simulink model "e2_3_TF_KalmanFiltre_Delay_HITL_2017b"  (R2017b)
settings: Solver=ode4  StartTime=0.0  StopTime=100  FixedStep=sampleTime  RelTol=1e-3  EnableMultiTasking=on
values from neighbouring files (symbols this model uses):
  k_d_x = 0.7    [startSimulation.m]
  k_d_y = 0.7    [startSimulation.m]
  k_d_yaw = 0.05    [startSimulation.m]
  k_d_z = 0.05    [startSimulation.m]
  k_i_x = 0.01    [startSimulation.m]
  k_i_y = 0.01    [startSimulation.m]
  k_i_yaw = 0.01    [startSimulation.m]
  k_i_z = 0.01    [startSimulation.m]
  k_p_x = 1    [startSimulation.m]
  k_p_y = 1    [startSimulation.m]
  k_p_yaw = 2    [startSimulation.m]
  k_p_z = 3    [startSimulation.m]
  saturation_psi = 2    [startSimulation.m]
  saturation_x = 2    [startSimulation.m]
  saturation_y = 2    [startSimulation.m]
  saturation_z = 2    [startSimulation.m]
undefined symbols (not defined in the file or in its folder): DiscIntNeverNeededParam, KiRollAttitude, sigbuilder_block
libraries: simulink x10, aerolibanimutils x2, etargetslib x2
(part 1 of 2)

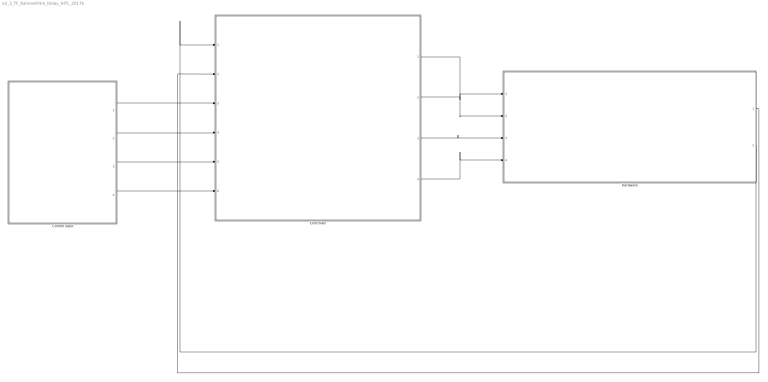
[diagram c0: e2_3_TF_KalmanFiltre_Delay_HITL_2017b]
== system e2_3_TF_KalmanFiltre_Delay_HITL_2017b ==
  Control Input : Subsystem
  "Controller " : Subsystem
  Hardware : Subsystem
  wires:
  "Controller "/1(Controller Output X) -> Hardware/1(X)
  "Controller "/2(Controller Output Y) -> Hardware/2(Y)
  "Controller "/3(Controller Output H) -> Hardware/3(H)
  "Controller "/4(Controller Output Psi) -> Hardware/4(Psi)
  Control Input/1(ux) -> "Controller "/3(Control input X)
  Control Input/2(uy) -> "Controller "/4(Control input Y)
  Control Input/3(uz) -> "Controller "/5(Control input H)
  Control Input/4(upsi) -> "Controller "/6(Control input Psi)
  Hardware/1(Vel) -> "Controller "/2(Feedback Velocity)
  Hardware/2(Pos) -> "Controller "/1(Feedback Position)

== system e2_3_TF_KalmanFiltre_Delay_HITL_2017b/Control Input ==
  Bloc Test Position Fixe : Subsystem
  Bus Creator : BusCreator  Inputs=4
  Demux : Demux
  Simulation Pace : aerolibanimutils/Simulation Pace  Commented=on  SimulationPace=100  SleepMode=MATLAB Thread  OutputPaceError=off  SampleTime=-1
  ux : Outport  VectorParamsAs1DForOutWhenUnconnected=off
  uy : Outport  Port=2  VectorParamsAs1DForOutWhenUnconnected=off
  uz : Outport  Port=3  VectorParamsAs1DForOutWhenUnconnected=off
  upsi : Outport  Port=4  VectorParamsAs1DForOutWhenUnconnected=off
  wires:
  Demux/2 -> uy/1
  Demux/1 -> ux/1
  Bloc Test Position Fixe/2(uy) -> Bus Creator/2
  Demux/3 -> uz/1
  Demux/4 -> upsi/1
  Bloc Test Position Fixe/4(upsi) -> Bus Creator/4
  Bloc Test Position Fixe/3(uz) -> Bus Creator/3
  Bloc Test Position Fixe/1(ux) -> Bus Creator/1
  Bus Creator/1 -> Demux/1

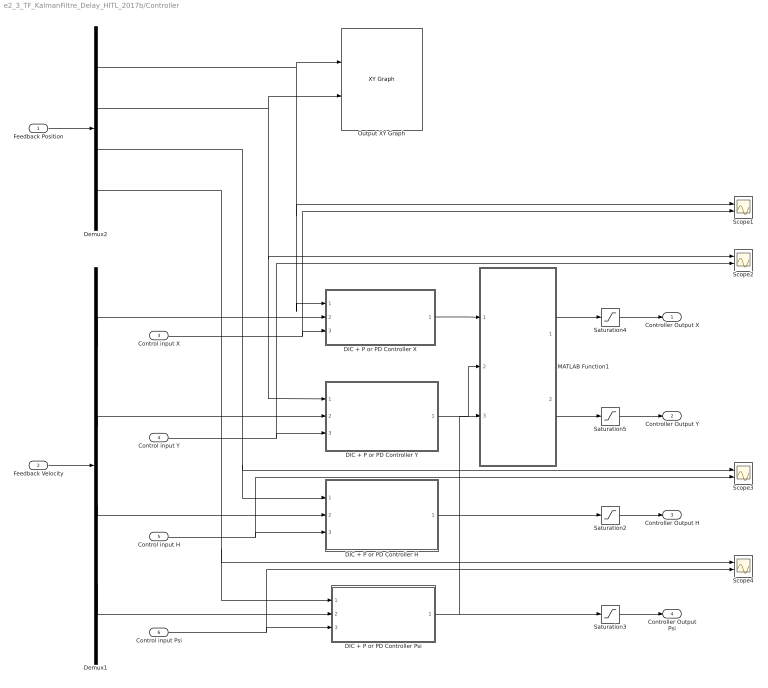
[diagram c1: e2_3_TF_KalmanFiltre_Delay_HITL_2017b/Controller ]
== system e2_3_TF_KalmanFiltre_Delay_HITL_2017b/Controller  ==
  Feedback Position : Inport
  Feedback Velocity : Inport  Port=2
  Control input X : Inport  Port=3
  Control input Y : Inport  Port=4
  Control input H : Inport  Port=5
  Control input Psi : Inport  Port=6
  DIC + P or PD Controller H : Subsystem
  DIC + P or PD Controller Psi : Subsystem
  DIC + P or PD Controller X : Subsystem
  DIC + P or PD Controller Y : Subsystem
  Demux1 : Demux
  Demux2 : Demux
  MATLAB Function1 : MATLAB Function  TreatAsAtomicUnit=on
  Output XY Graph : simulink/Sinks/XY Graph  Commented=on  xmin=-5  xmax=5  ymin=-5  ymax=5  st=-1
  Saturation2 : Saturate  UpperLimit=saturation_z  LowerLimit=-saturation_z
  Saturation3 : Saturate  UpperLimit=saturation_psi  LowerLimit=-saturation_psi
  Saturation4 : Saturate  UpperLimit=saturation_x  LowerLimit=-saturation_x
  Saturation5 : Saturate  UpperLimit=saturation_y  LowerLimit=-saturation_y
  Scope{1..4} (4 alike) : Scope  NumInputPorts=2
  Controller Output X : Outport  VectorParamsAs1DForOutWhenUnconnected=off
  Controller Output Y : Outport  Port=2  VectorParamsAs1DForOutWhenUnconnected=off
  Controller Output H : Outport  Port=3  VectorParamsAs1DForOutWhenUnconnected=off
  Controller Output Psi : Outport  Port=4  VectorParamsAs1DForOutWhenUnconnected=off
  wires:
  Feedback Position/1 -> Demux2/1
  Feedback Velocity/1 -> Demux1/1
  Demux1/2 -> DIC + P or PD Controller Y/2(Feedback Velocity Y)
  Demux2/3 -> Scope3/1, DIC + P or PD Controller H/1(Feedback Position H)
  Demux1/1 -> DIC + P or PD Controller X/2(Feedback Velocity X)
  Demux1/3 -> DIC + P or PD Controller H/2(Feedback Velocity H)
  Control input X/1 -> Scope1/2, DIC + P or PD Controller X/3(Control Input X)
  Control input H/1 -> Scope3/2, DIC + P or PD Controller H/3(Control Input H)
  Saturation4/1 -> Controller Output X/1
  Saturation5/1 -> Controller Output Y/1
  Saturation2/1 -> Controller Output H/1
  Saturation3/1 -> Controller Output Psi/1
  Control input Y/1 -> Scope2/2, DIC + P or PD Controller Y/3(Control Input Y)
  DIC + P or PD Controller H/1(Controller Output H) -> Saturation2/1
  DIC + P or PD Controller Psi/1(Controller Output Psi) -> MATLAB Function1/3(psi), Saturation3/1
  Demux2/1 -> Scope1/1, DIC + P or PD Controller X/1(Feedback Position X), Output XY Graph/1
  Demux2/2 -> Scope2/1, DIC + P or PD Controller Y/1(Feedback Position Y), Output XY Graph/2
  Demux2/4 -> Scope4/1, DIC + P or PD Controller Psi/1(Feedback Position Psi)
  Demux1/4 -> DIC + P or PD Controller Psi/2(Feedback Velocity Psi)
  Control input Psi/1 -> Scope4/2, DIC + P or PD Controller Psi/3(Control input Psi)
  MATLAB Function1/2(y) -> Saturation5/1
  MATLAB Function1/1(x) -> Saturation4/1
  DIC + P or PD Controller X/1(Controller Output X) -> MATLAB Function1/1(eax)
  DIC + P or PD Controller Y/1(Controller Output Y) -> MATLAB Function1/2(eay)

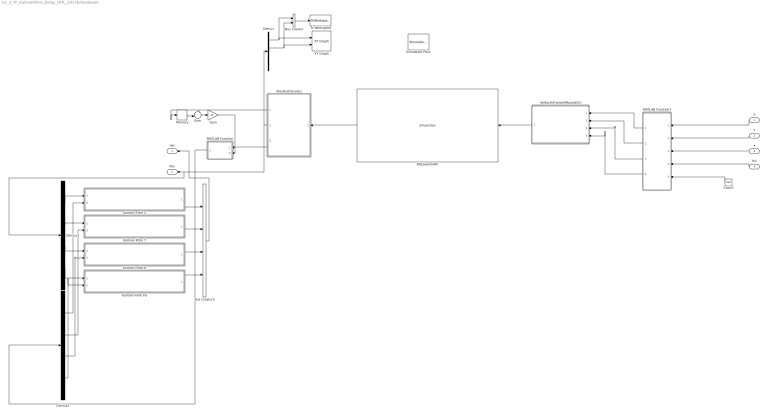
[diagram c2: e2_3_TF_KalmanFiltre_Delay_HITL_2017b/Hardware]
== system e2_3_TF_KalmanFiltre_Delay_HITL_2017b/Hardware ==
  X : Inport
  Y : Inport  Port=2
  H : Inport  Port=3
  Psi : Inport  Port=4
  Bus Creator : BusCreator  Inputs=2
  Bus Creator5 : BusCreator  Inputs=4
  Clock1 : Clock
  Demux : Demux
  Demux1 : Demux
  Demux2 : Demux
  Gain : Gain  Gain=25
  Kalman Filtre H : Subsystem
  Kalman Filtre Psi : Subsystem
  Kalman Filtre X : Subsystem
  Kalman Filtre Y : Subsystem
  MATLAB Function : MATLAB Function  TreatAsAtomicUnit=on
  MATLAB Function7 : MATLAB Function  TreatAsAtomicUnit=on
  MavOutDecode1 : MATLAB Function  TreatAsAtomicUnit=on
  Memory : Memory
  RflySwarmAPI : S-Function  FunctionName=RflyUdpFast  Parameters=port,num,modeValue,T,ip  SFunctionDeploymentMode=off  EnableBusSupport=off  mask(UDP Receive){ip=255.255.255.255, port=20100, num=1, mode=FullData Mode, T=1/25, modeValue=0}
      mask prompts: ip "UDP IP Address"; port "UDP Port"; num "vehicle Number"; mode "UDP Mode"; T "Sample Time"
      mask help: This block receives bytes from an UDP/IP connection. The first parameter is the UDP port on the first CopterSim App The second parameter is the total vehicle number The third parameter is the data mode. check the help button for the definition
      mask init:
      | if strcmp(mode,'FullData Mode')
      |     modeValue = 0;
      | elseif strcmp(mode,'SimpleData Mode') 
      |     modeValue = 1;
      | elseif strcmp(mode,'UltraSimple Mode') 
      |     modeValue = 2;
      | else
      |     modeValue = 0;
      | end
  Simulation Pace : aerolibanimutils/Simulation Pace  SimulationPace=1  SleepMode=MATLAB Thread  OutputPaceError=off  SampleTime=-1
  Sum : Sum  Inputs=+-|
  To Workspace : ToWorkspace  VariableName=Pos1  SaveFormat=Timeseries  SampleTime=-1
  VelEarthFrameOffboardCtrl : Subsystem
  XY Graph : simulink/Sinks/XY Graph  Commented=on  xmin=-1  xmax=1  ymin=-1  ymax=1  st=-1
  Vel : Outport  VectorParamsAs1DForOutWhenUnconnected=off
  Pos : Outport  Port=2  VectorParamsAs1DForOutWhenUnconnected=off
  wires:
  Gain/1 -> MATLAB Function/2(psi)
  Demux/2 -> Bus Creator/2, XY Graph/2
  Demux/1 -> Bus Creator/1, XY Graph/1
  Sum/1 -> Gain/1
  X/1 -> MATLAB Function7/1(X)
  MATLAB Function7/2(y1) -> VelEarthFrameOffboardCtrl/2(VeY_ms)
  MATLAB Function7/3(h1) -> VelEarthFrameOffboardCtrl/3(VeZ_ms)
  MATLAB Function7/1(x1) -> VelEarthFrameOffboardCtrl/1(VeX_ms)
  Clock1/1 -> MATLAB Function7/5(t)
  Memory/1 -> Sum/2
  MavOutDecode1/1(Psi) -> Memory/1, Sum/1
  RflySwarmAPI/1 -> MavOutDecode1/1(u)
  VelEarthFrameOffboardCtrl/1(Out1) -> RflySwarmAPI/1
  Bus Creator/1 -> To Workspace/1
  MavOutDecode1/3(localVel) -> MATLAB Function/1(v)
  MATLAB Function7/4(p1) -> VelEarthFrameOffboardCtrl/4(yawRate_rads)
  Y/1 -> MATLAB Function7/2(Y)
  H/1 -> MATLAB Function7/3(H)
  Psi/1 -> MATLAB Function7/4(Psi)
  Demux1/1 -> Kalman Filtre X/1(The system output: Position)
  Kalman Filtre X/1(Out velocity feedback) -> Bus Creator5/1
  MavOutDecode1/2(localPos) -> Demux1/1, Pos/1, Demux/1
  Kalman Filtre Psi/1(Out velocity feedback) -> Bus Creator5/4
  Demux2/2 -> Kalman Filtre Y/2(In2)
  Demux1/4 -> Kalman Filtre Psi/1(The system output: Position)
  Demux1/2 -> Kalman Filtre Y/1(The system output: Position)
  Demux2/4 -> Kalman Filtre Psi/2(In2)
  Demux1/3 -> Kalman Filtre H/1(The system output: Position)
  Demux2/1 -> Kalman Filtre X/2(In2)
  Kalman Filtre H/1(Out velocity feedback) -> Bus Creator5/3
  MATLAB Function/1(y) -> Demux2/1
  Demux2/3 -> Kalman Filtre H/2(In2)
  Kalman Filtre Y/1(Out velocity feedback) -> Bus Creator5/2
  Bus Creator5/1 -> Vel/1

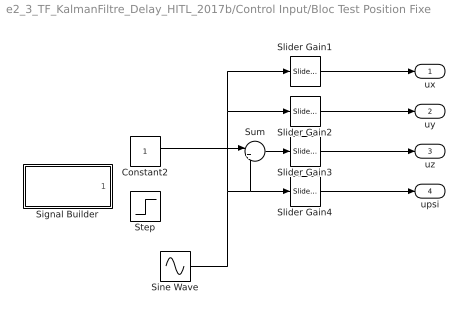
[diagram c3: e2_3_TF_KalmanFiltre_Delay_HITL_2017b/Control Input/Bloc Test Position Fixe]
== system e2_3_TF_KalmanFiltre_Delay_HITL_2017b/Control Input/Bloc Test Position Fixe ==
  Constant2 : Constant
  Signal Builder : Subsystem  Tag=STV Subsys  LoadFcn=sigbuilder_block('load');  StartFcn=sigbuilder_block('start');  StopFcn=sigbuilder_block('stop');  ClipboardFcn=sigbuilder_block('clipboard');  mask(Sigbuilder block){tuvar=[0:10]}
      mask help: Simulink:masks:SigbuilderBlock_MD
      mask init:
      | if ~strcmp(get_param(bdroot(gcbh),'SimulationStatus'),'stopped') tuvar = sigbuilder_block('maskInit'); end
  Sine Wave : Sin  Frequency=0.5  SampleTime=0
  Slider Gain1 : simulink/Math Operations/Slider Gain  gain=0  low=-10  high=10
  Slider Gain2 : simulink/Math Operations/Slider Gain  gain=0  low=-10  high=10
  Slider Gain3 : simulink/Math Operations/Slider Gain  gain=1  low=-2  high=2
  Slider Gain4 : simulink/Math Operations/Slider Gain  gain=0  low=-2  high=2
  Step : Step  Time=5  SampleTime=0
  Sum : Sum  Inputs=|++
  ux : Outport  VectorParamsAs1DForOutWhenUnconnected=off
  uy : Outport  Port=2  VectorParamsAs1DForOutWhenUnconnected=off
  uz : Outport  Port=3  VectorParamsAs1DForOutWhenUnconnected=off
  upsi : Outport  Port=4  VectorParamsAs1DForOutWhenUnconnected=off
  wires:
  Slider Gain1/1 -> ux/1
  Slider Gain2/1 -> uy/1
  Slider Gain3/1 -> uz/1
  Slider Gain4/1 -> upsi/1
  Constant2/1 -> Sum/1
  Sine Wave/1 -> Sum/2, Slider Gain4/1, Slider Gain2/1, Slider Gain1/1
  Sum/1 -> Slider Gain3/1

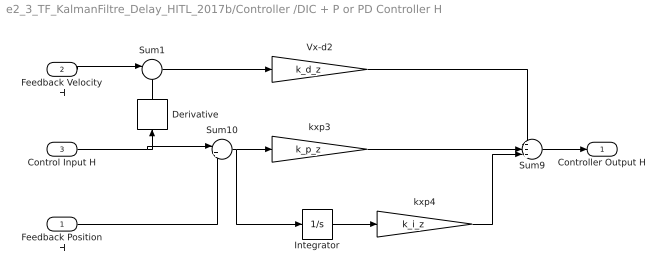
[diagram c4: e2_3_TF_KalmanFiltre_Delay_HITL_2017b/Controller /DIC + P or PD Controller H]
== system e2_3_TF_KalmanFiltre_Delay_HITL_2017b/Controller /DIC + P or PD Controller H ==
  Feedback Position H : Inport
  Feedback Velocity H : Inport  Port=2
  Control Input H : Inport  Port=3
  Derivative : Derivative
  Integrator : Integrator
  Sum1 : Sum  Inputs=|-+
  Sum10 : Sum  Inputs=|+-
  Sum9 : Sum  Inputs=+++|
  Vx-d2 : Gain  Gain=k_d_z
  kxp3 : Gain  Gain=k_p_z
  kxp4 : Gain  Gain=k_i_z
  Controller Output H : Outport  VectorParamsAs1DForOutWhenUnconnected=off
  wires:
  Sum9/1 -> Controller Output H/1
  Sum10/1 -> kxp3/1, Integrator/1
  kxp3/1 -> Sum9/2
  Vx-d2/1 -> Sum9/1
  Feedback Velocity H/1 -> Sum1/1
  Sum1/1 -> Vx-d2/1
  Integrator/1 -> kxp4/1
  kxp4/1 -> Sum9/3
  Control Input H/1 -> Sum10/1, Derivative/1
  Feedback Position H/1 -> Sum10/2
  Derivative/1 -> Sum1/2

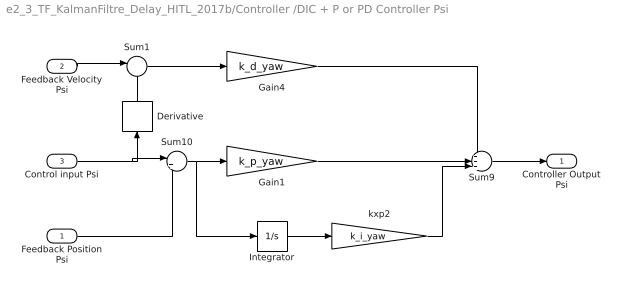
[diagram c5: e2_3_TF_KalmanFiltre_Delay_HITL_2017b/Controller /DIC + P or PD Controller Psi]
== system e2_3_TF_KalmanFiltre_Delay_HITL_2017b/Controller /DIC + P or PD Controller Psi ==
  Feedback Position Psi : Inport
  Feedback Velocity Psi : Inport  Port=2
  Control input Psi : Inport  Port=3
  Derivative : Derivative
  Gain1 : Gain  Gain=k_p_yaw
  Gain4 : Gain  Gain=k_d_yaw
  Integrator : Integrator
  Sum1 : Sum  Inputs=|-+
  Sum10 : Sum  Inputs=|+-
  Sum9 : Sum  Inputs=+++|
  kxp2 : Gain  Gain=k_i_yaw
  Controller Output Psi : Outport  VectorParamsAs1DForOutWhenUnconnected=off
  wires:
  Sum9/1 -> Controller Output Psi/1
  kxp2/1 -> Sum9/3
  Control input Psi/1 -> Sum10/1, Derivative/1
  Gain4/1 -> Sum9/1
  Sum10/1 -> Gain1/1, Integrator/1
  Integrator/1 -> kxp2/1
  Feedback Velocity Psi/1 -> Sum1/1
  Sum1/1 -> Gain4/1
  Gain1/1 -> Sum9/2
  Derivative/1 -> Sum1/2
  Feedback Position Psi/1 -> Sum10/2

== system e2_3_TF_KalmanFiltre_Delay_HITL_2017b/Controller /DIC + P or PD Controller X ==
  Feedback Position X : Inport
  Feedback Velocity X : Inport  Port=2
  Control Input X : Inport  Port=3
  PID1 : Subsystem
  Sum3 : Sum  Inputs=|+-
  Sum4 : Sum  Inputs=|+-
  roll_attitude2 : simulink/Continuous/PID Controller  Controller=P  Form=Parallel  TimeDomain=Discrete-time  SampleTime=-1  IntegratorMethod=Forward Euler  FilterMethod=Forward Euler  ControllerParametersSource=internal  P=1  I=KiRollAttitude  D=0.01  UseFilter=on  N=100  TunerSelectOption=Transfer Function Based (PID Tuner App)  InitialConditionSource=internal  InitialConditionForIntegrator=0  InitialConditionForFilter=0  DifferentiatorICPrevScaledInput=0  ExternalReset=none  TrackingMode=off  Kt=1  LimitOutput=on  UpperSaturationLimit=100  LowerSaturationLimit=-100  LinearizeAsGain=on  AntiWindupMode=back-calculation  Kb=1  POutMin=[]  POutMax=[]  IOutMin=[]  IOutMax=[]  DOutMin=[]  DOutMax=[]  NOutMin=[]  NOutMax=[]  SumOutMin=[]  SumOutMax=[]  SaturationOutMin=[]  SaturationOutMax=[]  PParamMin=[]  PParamMax=[]  IParamMin=[]  IParamMax=[]  DParamMin=[]  DParamMax=[]  NParamMin=[]  NParamMax=[]  KbParamMin=[]  KbParamMax=[]  KtParamMin=[]  KtParamMax=[]  KbOutMin=[]  KbOutMax=[]  KtOutMin=[]  KtOutMax=[]  IntegratorOutMin=[]  IntegratorOutMax=[]  FilterOutMin=[]  FilterOutMax=[]  SumI1OutMin=[]  SumI1OutMax=[]  SumI2OutMin=[]  SumI2OutMax=[]  SumI3OutMin=[]  SumI3OutMax=[]  SumDOutMin=[]  SumDOutMax=[]  DifferentiatorOutMin=[]  DifferentiatorOutMax=[]  FilterDiffOutCoefMin=[]  FilterDiffOutCoefMax=[]  ReciprocalOutMin=[]  ReciprocalOutMax=[]  SumDenOutMin=[]  SumDenOutMax=[]  SumNumOutMin=[]  SumNumOutMax=[]  DivideOutMin=[]  DivideOutMax=[]  IntegratorContinuousStateAttributes=''  IntegratorStateMustResolveToSignalObject=off  IntegratorRTWStateStorageClass=Auto  FilterContinuousStateAttributes=''  FilterStateMustResolveToSignalObject=off  FilterRTWStateStorageClass=Auto  InitialConditionSetting=State (most efficient)
  Controller Output X : Outport  VectorParamsAs1DForOutWhenUnconnected=off
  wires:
  roll_attitude2/1 -> Sum4/1
  Sum3/1 -> roll_attitude2/1
  Sum4/1 -> PID1/1(x)
  PID1/1(y) -> Controller Output X/1
  Feedback Velocity X/1 -> Sum4/2
  Control Input X/1 -> Sum3/1
  Feedback Position X/1 -> Sum3/2

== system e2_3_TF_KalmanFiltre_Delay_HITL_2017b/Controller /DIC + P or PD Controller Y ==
  Feedback Position Y : Inport
  Feedback Velocity Y : Inport  Port=2
  Control Input Y : Inport  Port=3
  PID2 : Subsystem
  Sum : Sum  Inputs=|+-
  Sum2 : Sum  Inputs=|+-
  roll_attitude : simulink/Continuous/PID Controller  Controller=P  Form=Parallel  TimeDomain=Discrete-time  SampleTime=-1  IntegratorMethod=Forward Euler  FilterMethod=Forward Euler  ControllerParametersSource=internal  P=1  I=KiRollAttitude  D=0.01  UseFilter=on  N=100  TunerSelectOption=Transfer Function Based (PID Tuner App)  InitialConditionSource=internal  InitialConditionForIntegrator=0  InitialConditionForFilter=0  DifferentiatorICPrevScaledInput=0  ExternalReset=none  TrackingMode=off  Kt=1  LimitOutput=on  UpperSaturationLimit=1  LowerSaturationLimit=-1  LinearizeAsGain=on  AntiWindupMode=back-calculation  Kb=1  POutMin=[]  POutMax=[]  IOutMin=[]  IOutMax=[]  DOutMin=[]  DOutMax=[]  NOutMin=[]  NOutMax=[]  SumOutMin=[]  SumOutMax=[]  SaturationOutMin=[]  SaturationOutMax=[]  PParamMin=[]  PParamMax=[]  IParamMin=[]  IParamMax=[]  DParamMin=[]  DParamMax=[]  NParamMin=[]  NParamMax=[]  KbParamMin=[]  KbParamMax=[]  KtParamMin=[]  KtParamMax=[]  KbOutMin=[]  KbOutMax=[]  KtOutMin=[]  KtOutMax=[]  IntegratorOutMin=[]  IntegratorOutMax=[]  FilterOutMin=[]  FilterOutMax=[]  SumI1OutMin=[]  SumI1OutMax=[]  SumI2OutMin=[]  SumI2OutMax=[]  SumI3OutMin=[]  SumI3OutMax=[]  SumDOutMin=[]  SumDOutMax=[]  DifferentiatorOutMin=[]  DifferentiatorOutMax=[]  FilterDiffOutCoefMin=[]  FilterDiffOutCoefMax=[]  ReciprocalOutMin=[]  ReciprocalOutMax=[]  SumDenOutMin=[]  SumDenOutMax=[]  SumNumOutMin=[]  SumNumOutMax=[]  DivideOutMin=[]  DivideOutMax=[]  IntegratorContinuousStateAttributes=''  IntegratorStateMustResolveToSignalObject=off  IntegratorRTWStateStorageClass=Auto  FilterContinuousStateAttributes=''  FilterStateMustResolveToSignalObject=off  FilterRTWStateStorageClass=Auto  InitialConditionSetting=State (most efficient)
  Controller Output Y : Outport  VectorParamsAs1DForOutWhenUnconnected=off
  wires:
  Sum/1 -> roll_attitude/1
  roll_attitude/1 -> Sum2/1
  Sum2/1 -> PID2/1(x)
  Feedback Position Y/1 -> Sum/2
  Feedback Velocity Y/1 -> Sum2/2
  Control Input Y/1 -> Sum/1
  PID2/1(y) -> Controller Output Y/1

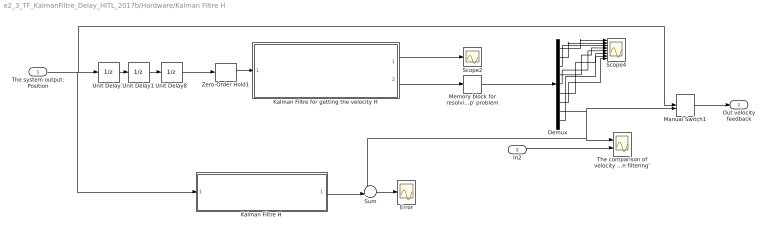
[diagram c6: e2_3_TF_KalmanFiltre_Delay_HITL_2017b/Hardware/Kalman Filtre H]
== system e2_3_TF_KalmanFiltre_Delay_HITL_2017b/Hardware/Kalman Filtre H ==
  The system output: Position : Inport
  In2 : Inport  Port=2
  Demux : Demux  Outputs=9
  Error : Scope
  Kalman Filtre H : Subsystem
  Kalman Filtre for getting the velocity H : MATLAB Function  TreatAsAtomicUnit=on
  Manual Switch1 : ManualSwitch  CurrentSetting=0
  Memory block for resolving the 'algebraic loop' problem : Memory
  Scope2 : Scope
  Scope4 : Scope  NumInputPorts=8
  Sum : Sum  Inputs=-+|
  The comparison of velocity signal between 'Derivative' and 'Kalman filtering' : Scope  NumInputPorts=2
  Unit Delay1 : UnitDelay  SampleTime=-1  HasFrameUpgradeWarning=on
  Unit Delay7 : UnitDelay  SampleTime=-1  HasFrameUpgradeWarning=on
  Unit Delay8 : UnitDelay  SampleTime=-1  HasFrameUpgradeWarning=on
  Zero-Order Hold1 : ZeroOrderHold  SampleTime=-1
  Out velocity feedback : Outport  VectorParamsAs1DForOutWhenUnconnected=off
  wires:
  Kalman Filtre for getting the velocity H/1(Covariance_matrice) -> Scope2/1
  Kalman Filtre for getting the velocity H/2(X_Kalmanfiltred) -> Memory block for resolving the 'algebraic loop' problem/1
  Memory block for resolving the 'algebraic loop' problem/1 -> Demux/1
  Zero-Order Hold1/1 -> Kalman Filtre for getting the velocity H/1(Mesurement_Velocity)
  Manual Switch1/1 -> Out velocity feedback/1
  Demux/1 -> Scope4/1
  The system output: Position/1 -> Kalman Filtre H/1(The system output: Position), Manual Switch1/1, Unit Delay7/1
  Demux/2 -> Scope4/2
  Demux/3 -> Scope4/3
  Demux/4 -> Scope4/4
  Demux/5 -> Scope4/5
  Unit Delay8/1 -> Zero-Order Hold1/1
  Demux/6 -> Scope4/6
  Demux/7 -> Scope4/8
  Demux/8 -> Sum/1, The comparison of velocity signal between 'Derivative' and 'Kalman filtering'/1, Manual Switch1/2
  Demux/9 -> Scope4/7
  In2/1 -> The comparison of velocity signal between 'Derivative' and 'Kalman filtering'/2
  Unit Delay7/1 -> Unit Delay1/1
  Unit Delay1/1 -> Unit Delay8/1
  Sum/1 -> Error/1
  Kalman Filtre H/1(Out velocity feedback) -> Sum/2

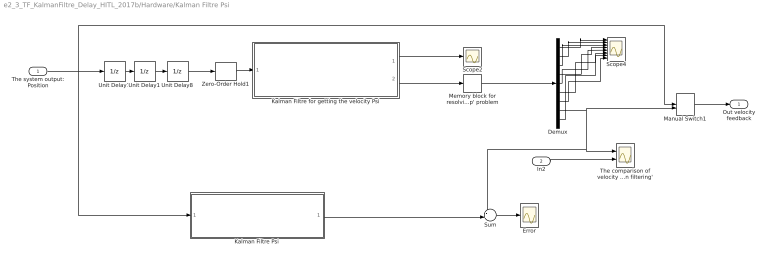
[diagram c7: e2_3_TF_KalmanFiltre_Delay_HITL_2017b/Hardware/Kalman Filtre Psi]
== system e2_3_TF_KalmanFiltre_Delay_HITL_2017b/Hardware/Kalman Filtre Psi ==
  The system output: Position : Inport
  In2 : Inport  Port=2
  Demux : Demux  Outputs=9
  Error : Scope
  Kalman Filtre Psi : Subsystem
  Kalman Filtre for getting the velocity Psi : MATLAB Function  TreatAsAtomicUnit=on
  Manual Switch1 : ManualSwitch  CurrentSetting=0
  Memory block for resolving the 'algebraic loop' problem : Memory
  Scope2 : Scope
  Scope4 : Scope  NumInputPorts=8
  Sum : Sum  Inputs=-+|
  The comparison of velocity signal between 'Derivative' and 'Kalman filtering' : Scope  NumInputPorts=2
  Unit Delay1 : UnitDelay  SampleTime=-1  HasFrameUpgradeWarning=on
  Unit Delay7 : UnitDelay  SampleTime=-1  HasFrameUpgradeWarning=on
  Unit Delay8 : UnitDelay  SampleTime=-1  HasFrameUpgradeWarning=on
  Zero-Order Hold1 : ZeroOrderHold  SampleTime=-1
  Out velocity feedback : Outport  VectorParamsAs1DForOutWhenUnconnected=off
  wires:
  Kalman Filtre for getting the velocity Psi/1(Covariance_matrice) -> Scope2/1
  Kalman Filtre for getting the velocity Psi/2(X_Kalmanfiltred) -> Memory block for resolving the 'algebraic loop' problem/1
  Memory block for resolving the 'algebraic loop' problem/1 -> Demux/1
  Zero-Order Hold1/1 -> Kalman Filtre for getting the velocity Psi/1(Mesurement_Velocity)
  Manual Switch1/1 -> Out velocity feedback/1
  Demux/1 -> Scope4/1
  The system output: Position/1 -> Kalman Filtre Psi/1(The system output: Position), Manual Switch1/1, Unit Delay7/1
  Demux/2 -> Scope4/2
  Demux/3 -> Scope4/3
  Demux/4 -> Scope4/4
  Demux/5 -> Scope4/5
  Unit Delay8/1 -> Zero-Order Hold1/1
  Demux/6 -> Scope4/6
  Demux/7 -> Scope4/8
  Demux/8 -> Sum/1, The comparison of velocity signal between 'Derivative' and 'Kalman filtering'/1, Manual Switch1/2
  Demux/9 -> Scope4/7
  In2/1 -> The comparison of velocity signal between 'Derivative' and 'Kalman filtering'/2
  Unit Delay7/1 -> Unit Delay1/1
  Unit Delay1/1 -> Unit Delay8/1
  Sum/1 -> Error/1
  Kalman Filtre Psi/1(Out velocity feedback) -> Sum/2

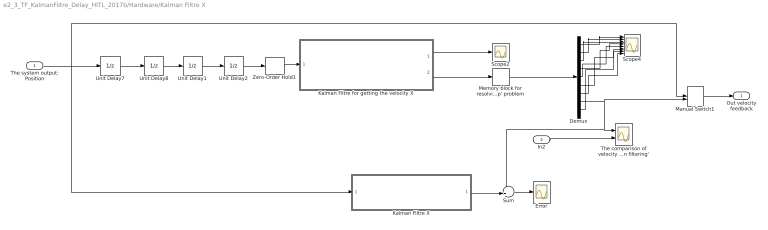
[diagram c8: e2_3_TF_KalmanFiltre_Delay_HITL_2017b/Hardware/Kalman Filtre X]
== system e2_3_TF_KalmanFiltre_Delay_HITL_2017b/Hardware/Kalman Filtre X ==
  The system output: Position : Inport
  In2 : Inport  Port=2
  Demux : Demux  Outputs=9
  Error : Scope
  Kalman Filtre X : Subsystem
  Kalman Filtre for getting the velocity X : MATLAB Function  TreatAsAtomicUnit=on
  Manual Switch1 : ManualSwitch  CurrentSetting=0
  Memory block for resolving the 'algebraic loop' problem : Memory  InheritSampleTime=on
  Scope2 : Scope
  Scope4 : Scope  NumInputPorts=8
  Sum : Sum  Inputs=-+|
  The comparison of velocity signal between 'Derivative' and 'Kalman filtering' : Scope  NumInputPorts=2
  Unit Delay{1..2,7..8} (4 alike) : UnitDelay  SampleTime=-1  HasFrameUpgradeWarning=on
  Zero-Order Hold1 : ZeroOrderHold  SampleTime=-1
  Out velocity feedback : Outport  VectorParamsAs1DForOutWhenUnconnected=off
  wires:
  Kalman Filtre for getting the velocity X/1(Covariance_matrice) -> Scope2/1
  Kalman Filtre for getting the velocity X/2(X_Kalmanfiltred) -> Memory block for resolving the 'algebraic loop' problem/1
  Memory block for resolving the 'algebraic loop' problem/1 -> Demux/1
  Zero-Order Hold1/1 -> Kalman Filtre for getting the velocity X/1(Mesurement_Velocity)
  Manual Switch1/1 -> Out velocity feedback/1
  Demux/1 -> Scope4/1
  The system output: Position/1 -> Kalman Filtre X/1(The system output: Position), Manual Switch1/1, Unit Delay7/1
  Demux/2 -> Scope4/2
  Demux/3 -> Scope4/3
  Demux/4 -> Scope4/4
  Demux/5 -> Scope4/5
  Unit Delay7/1 -> Unit Delay8/1
  Unit Delay8/1 -> Unit Delay1/1
  Demux/6 -> Scope4/6
  Demux/7 -> Scope4/8
  Demux/8 -> Sum/1, The comparison of velocity signal between 'Derivative' and 'Kalman filtering'/1, Manual Switch1/2
  Demux/9 -> Scope4/7
  In2/1 -> The comparison of velocity signal between 'Derivative' and 'Kalman filtering'/2
  Unit Delay1/1 -> Unit Delay2/1
  Unit Delay2/1 -> Zero-Order Hold1/1
  Kalman Filtre X/1(Out velocity feedback) -> Sum/2
  Sum/1 -> Error/1

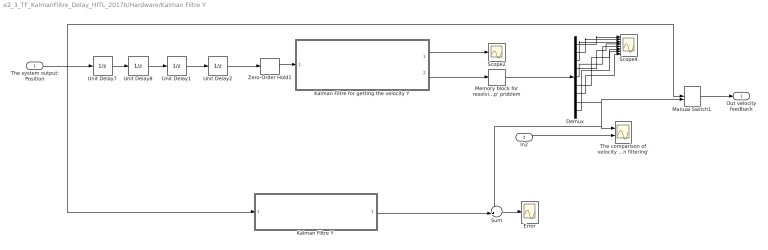
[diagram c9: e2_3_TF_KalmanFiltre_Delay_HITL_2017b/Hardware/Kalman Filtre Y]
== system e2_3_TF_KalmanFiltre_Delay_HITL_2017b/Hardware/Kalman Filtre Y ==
  The system output: Position : Inport
  In2 : Inport  Port=2
  Demux : Demux  Outputs=9
  Error : Scope
  Kalman Filtre Y : Subsystem
  Kalman Filtre for getting the velocity Y : MATLAB Function  TreatAsAtomicUnit=on
  Manual Switch1 : ManualSwitch  CurrentSetting=0
  Memory block for resolving the 'algebraic loop' problem : Memory
  Scope2 : Scope
  Scope4 : Scope  NumInputPorts=8
  Sum : Sum  Inputs=-+|
  The comparison of velocity signal between 'Derivative' and 'Kalman filtering' : Scope  NumInputPorts=2
  Unit Delay{1..2,7..8} (4 alike) : UnitDelay  SampleTime=-1  HasFrameUpgradeWarning=on
  Zero-Order Hold1 : ZeroOrderHold  SampleTime=-1
  Out velocity feedback : Outport  VectorParamsAs1DForOutWhenUnconnected=off
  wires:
  Kalman Filtre for getting the velocity Y/1(Covariance_matrice) -> Scope2/1
  Kalman Filtre for getting the velocity Y/2(X_Kalmanfiltred) -> Memory block for resolving the 'algebraic loop' problem/1
  Memory block for resolving the 'algebraic loop' problem/1 -> Demux/1
  Zero-Order Hold1/1 -> Kalman Filtre for getting the velocity Y/1(Mesurement_Velocity)
  Manual Switch1/1 -> Out velocity feedback/1
  Demux/1 -> Scope4/1
  The system output: Position/1 -> Kalman Filtre Y/1(The system output: Position), Unit Delay7/1, Manual Switch1/1
  Demux/2 -> Scope4/2
  Demux/3 -> Scope4/3
  Demux/4 -> Scope4/4
  Demux/5 -> Scope4/5
  Unit Delay2/1 -> Zero-Order Hold1/1
  Demux/6 -> Scope4/6
  Demux/7 -> Scope4/8
  Demux/8 -> Sum/1, The comparison of velocity signal between 'Derivative' and 'Kalman filtering'/1, Manual Switch1/2
  Demux/9 -> Scope4/7
  In2/1 -> The comparison of velocity signal between 'Derivative' and 'Kalman filtering'/2
  Unit Delay1/1 -> Unit Delay2/1
  Unit Delay8/1 -> Unit Delay1/1
  Unit Delay7/1 -> Unit Delay8/1
  Sum/1 -> Error/1
  Kalman Filtre Y/1(Out velocity feedback) -> Sum/2

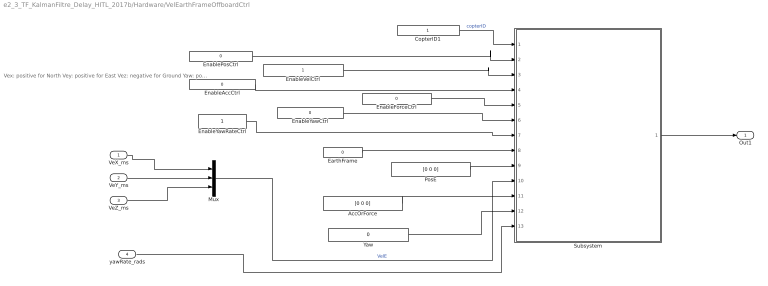
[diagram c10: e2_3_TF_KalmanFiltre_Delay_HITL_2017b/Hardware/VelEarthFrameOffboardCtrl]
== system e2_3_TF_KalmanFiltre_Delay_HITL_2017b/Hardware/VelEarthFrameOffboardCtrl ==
  note: Vex: positive for North Vey: positive for East Vez: negative for Ground Yaw: positive for right rotation
  VeX_ms : Inport
  VeY_ms : Inport  Port=2
  VeZ_ms : Inport  Port=3
  yawRate_rads : Inport  Port=4  PortDimensions=1
  AccOrForce : Constant  Value=[0 0 0]
  CopterID1 : Constant
  EarthFrame : Constant  Value=0
  EnableAccCtrl : Constant  Value=0
  EnableForceCtrl : Constant  Value=0
  EnablePosCtrl : Constant  Value=0
  EnableVelCtrl : Constant
  EnableYawCtrl : Constant  Value=0
  EnableYawRateCtrl : Constant
  Mux : Mux  Inputs=3
  PosE : Constant  Value=[0 0 0]
  Subsystem : Subsystem
  Yaw : Constant  Value=0
  Out1 : Outport
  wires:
  Yaw/1 -> Subsystem/12(yaw)
  EnableYawRateCtrl/1 -> Subsystem/7(EnYawrate)
  EnableYawCtrl/1 -> Subsystem/6(enYaw)
  EnableAccCtrl/1 -> Subsystem/4(enAcc)
  Mux/1 -> Subsystem/10(vel)  "VelE"
  EarthFrame/1 -> Subsystem/8(FrameIndex)
  yawRate_rads/1 -> Subsystem/13(yawrate)
  AccOrForce/1 -> Subsystem/11(acc)
  EnableVelCtrl/1 -> Subsystem/3(enVel)
  EnableForceCtrl/1 -> Subsystem/5(enForce)
  CopterID1/1 -> Subsystem/1(CopterID)  "copterID"
  EnablePosCtrl/1 -> Subsystem/2(enPos)
  PosE/1 -> Subsystem/9(pos)
  VeY_ms/1 -> Mux/2
  VeX_ms/1 -> Mux/1
  VeZ_ms/1 -> Mux/3
  Subsystem/1(Out1) -> Out1/1

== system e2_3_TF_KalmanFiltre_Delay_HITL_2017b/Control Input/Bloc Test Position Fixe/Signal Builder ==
  Demux : Demux  Tag=STV Demux  Outputs=1
  FromWs : FromWorkspace  Tag=STV FromWs  VariableName=tuvar
  Signal 2 : Outport  Tag=STV Outport  VectorParamsAs1DForOutWhenUnconnected=off
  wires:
  FromWs/1 -> Demux/1
  Demux/1 -> Signal 2/1

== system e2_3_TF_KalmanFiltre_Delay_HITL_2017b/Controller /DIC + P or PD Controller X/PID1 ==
  x : Inport
  Discrete Derivative : simulink/Discrete/Discrete Derivative  gainval=1.0  ICPrevScaledInput=0.0  OutMin=-5  OutMax=5  OutDataType=fixdt(1, 16)  OutScaling=2^-10  DoSatur=off
  Discrete-Time Integrator : DiscreteIntegrator  InitialConditionSetting=State (most efficient)  SampleTime=-1  LimitOutput=on  UpperSaturationLimit=5  LowerSaturationLimit=-5  ICPrevOutput=DiscIntNeverNeededParam  ICPrevScaledInput=DiscIntNeverNeededParam
  Sum : Sum  Inputs=+++  OutMin=-10  OutMax=10
  Vx-d3 : Gain  Gain=k_d_x
  kxp2 : Gain  Gain=k_i_x
  kxp3 : Gain  Gain=k_p_x
  y : Outport  InitialOutput=0  VectorParamsAs1DForOutWhenUnconnected=off
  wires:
  x/1 -> Vx-d3/1, kxp2/1, kxp3/1
  kxp2/1 -> Discrete-Time Integrator/1
  Vx-d3/1 -> Discrete Derivative/1
  kxp3/1 -> Sum/1
  Sum/1 -> y/1
  Discrete Derivative/1 -> Sum/3
  Discrete-Time Integrator/1 -> Sum/2

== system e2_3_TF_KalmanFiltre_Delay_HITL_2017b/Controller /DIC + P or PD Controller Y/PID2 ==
  x : Inport
  Discrete Derivative : simulink/Discrete/Discrete Derivative  gainval=1.0  ICPrevScaledInput=0.0  OutMin=[]  OutMax=[]  OutDataType=fixdt(1, 16)  OutScaling=2^-10  DoSatur=off
  Discrete-Time Integrator : DiscreteIntegrator  InitialConditionSetting=State (most efficient)  SampleTime=-1  LimitOutput=on  UpperSaturationLimit=10  LowerSaturationLimit=-10  ICPrevOutput=DiscIntNeverNeededParam  ICPrevScaledInput=DiscIntNeverNeededParam
  Sum : Sum  Inputs=+++  OutMin=-10  OutMax=10
  Vx-d2 : Gain  Gain=k_d_y
  kxp2 : Gain  Gain=k_p_y
  kxp3 : Gain  Gain=k_i_y
  y : Outport  InitialOutput=0  VectorParamsAs1DForOutWhenUnconnected=off
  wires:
  x/1 -> kxp2/1, kxp3/1, Vx-d2/1
  kxp3/1 -> Discrete-Time Integrator/1
  Vx-d2/1 -> Discrete Derivative/1
  kxp2/1 -> Sum/1
  Sum/1 -> y/1
  Discrete Derivative/1 -> Sum/3
  Discrete-Time Integrator/1 -> Sum/2

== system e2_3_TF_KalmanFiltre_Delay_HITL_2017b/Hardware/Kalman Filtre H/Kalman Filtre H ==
  The system output: Position : Inport
  Demux : Demux  Outputs=3
  Kalman Filtre for getting the velocity H : MATLAB Function  TreatAsAtomicUnit=on
  Memory block for resolving the 'algebraic loop' problem : Memory
  Scope2 : Scope
  Scope4 : Scope  NumInputPorts=2
  Out velocity feedback : Outport  VectorParamsAs1DForOutWhenUnconnected=off
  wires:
  Demux/2 -> Out velocity feedback/1
  Memory block for resolving the 'algebraic loop' problem/1 -> Demux/1
  Kalman Filtre for getting the velocity H/1(Covariance_matrice) -> Scope2/1
  The system output: Position/1 -> Kalman Filtre for getting the velocity H/1(Mesurement_Velocity)
  Demux/1 -> Scope4/1
  Kalman Filtre for getting the velocity H/2(X_Kalmanfiltred) -> Memory block for resolving the 'algebraic loop' problem/1
  Demux/3 -> Scope4/2

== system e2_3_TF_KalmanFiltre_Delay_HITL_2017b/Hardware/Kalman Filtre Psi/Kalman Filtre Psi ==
  The system output: Position : Inport
  Demux : Demux  Outputs=3
  Kalman Filtre for getting the velocity Psi : MATLAB Function  TreatAsAtomicUnit=on
  Memory block for resolving the 'algebraic loop' problem : Memory
  Scope1 : Scope  NumInputPorts=2
  Scope2 : Scope
  Out velocity feedback : Outport  VectorParamsAs1DForOutWhenUnconnected=off
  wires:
  Demux/2 -> Out velocity feedback/1
  Kalman Filtre for getting the velocity Psi/1(Covariance_matrice) -> Scope2/1
  The system output: Position/1 -> Kalman Filtre for getting the velocity Psi/1(Mesurement_Velocity)
  Demux/1 -> Scope1/1
  Demux/3 -> Scope1/2
  Kalman Filtre for getting the velocity Psi/2(X_Kalmanfiltred) -> Memory block for resolving the 'algebraic loop' problem/1
  Memory block for resolving the 'algebraic loop' problem/1 -> Demux/1

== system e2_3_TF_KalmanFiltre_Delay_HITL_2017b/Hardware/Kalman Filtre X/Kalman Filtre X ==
  The system output: Position : Inport
  Demux : Demux  Outputs=3
  Kalman Filtre for getting the velocity X : MATLAB Function  TreatAsAtomicUnit=on
  Memory block for resolving the 'algebraic loop' problem : Memory
  Scope2 : Scope
  Scope4 : Scope  NumInputPorts=2
  Out velocity feedback : Outport  VectorParamsAs1DForOutWhenUnconnected=off
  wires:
  Kalman Filtre for getting the velocity X/1(Covariance_matrice) -> Scope2/1
  Kalman Filtre for getting the velocity X/2(X_Kalmanfiltred) -> Memory block for resolving the 'algebraic loop' problem/1
  Memory block for resolving the 'algebraic loop' problem/1 -> Demux/1
  The system output: Position/1 -> Kalman Filtre for getting the velocity X/1(Mesurement_Velocity)
  Demux/2 -> Out velocity feedback/1
  Demux/1 -> Scope4/2
  Demux/3 -> Scope4/1

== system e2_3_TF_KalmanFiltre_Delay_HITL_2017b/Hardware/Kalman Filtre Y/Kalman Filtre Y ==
  The system output: Position : Inport
  Demux : Demux  Outputs=3
  Kalman Filtre for getting the velocity Y : MATLAB Function  TreatAsAtomicUnit=on
  Memory block for resolving the 'algebraic loop' problem : Memory
  Scope2 : Scope
  Scope4 : Scope  NumInputPorts=2
  Out velocity feedback : Outport  VectorParamsAs1DForOutWhenUnconnected=off
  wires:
  Kalman Filtre for getting the velocity Y/2(X_Kalmanfiltred) -> Memory block for resolving the 'algebraic loop' problem/1
  Demux/2 -> Out velocity feedback/1
  Kalman Filtre for getting the velocity Y/1(Covariance_matrice) -> Scope2/1
  Memory block for resolving the 'algebraic loop' problem/1 -> Demux/1
  The system output: Position/1 -> Kalman Filtre for getting the velocity Y/1(Mesurement_Velocity)
  Demux/1 -> Scope4/1
  Demux/3 -> Scope4/2

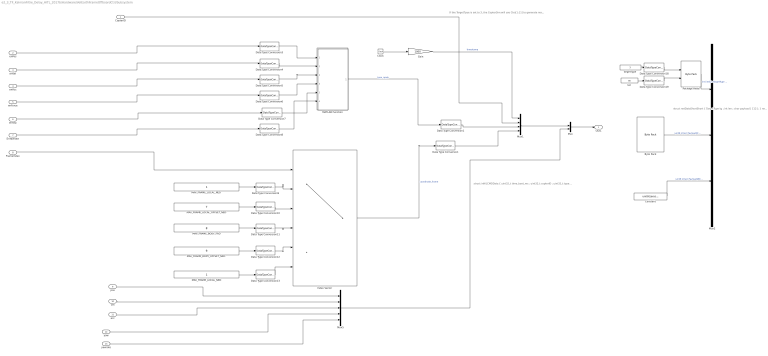
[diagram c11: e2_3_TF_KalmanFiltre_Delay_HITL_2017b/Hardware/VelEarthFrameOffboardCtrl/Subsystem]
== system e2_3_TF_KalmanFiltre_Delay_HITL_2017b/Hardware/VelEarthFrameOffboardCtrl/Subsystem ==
  note: struct netDataShortShort { TargetType tg ; int len ; char payload [ 112 ]; } netDataShortShort ;
  note: struct inHILCMDData { uint32_t time_boot_ms ; uint32_t copterID ; uint32_t type_mask ; uint32_t coordinate_frame ; float ctrls [ 11 ]; };
  note: If the TargetTpye is set to 3, the CopterSim will use Ctrs[1:11] to generate mavlink S ET_POSITION_TARGET_LOCAL_NED msg to UAV's Offboard mode Control， If the PX4 is not armed, CopterSim will send the arm command repeatly. If the PX4 is not in Offboard(Guided) Mode, CopterSim will send SET_MODE msg repeatly.
  CopterID : Inport
  enPos : Inport  Port=2
  enVel : Inport  Port=3
  enAcc : Inport  Port=4
  enForce : Inport  Port=5
  enYaw : Inport  Port=6
  EnYawrate : Inport  Port=7
  FrameIndex : Inport  Port=8
  pos : Inport  Port=9  PortDimensions=3
  vel : Inport  Port=10  PortDimensions=3
  acc : Inport  Port=11  PortDimensions=3
  yaw : Inport  Port=12  PortDimensions=1
  yawrate : Inport  Port=13  PortDimensions=1
  Byte Pack : etargetslib/Byte Pack  Commented=on  datatypes={'uint32','single'}  byteAlign=1
  Clock : Clock
  Constant : Constant  Commented=on  Value=uint8(zeros(32,1))
  Data Type Conversion : DataTypeConversion  OutDataTypeStr=double
  Data Type Conversion1 : DataTypeConversion  OutDataTypeStr=double
  Data Type Conversion{9..13} (5 alike) : DataTypeConversion  OutDataTypeStr=uint8
  Data Type Conversion18 : DataTypeConversion  Commented=on  OutDataTypeStr=uint32
  Data Type Conversion19 : DataTypeConversion  Commented=on  OutDataTypeStr=int32
  Data Type Conversion{3..8} (6 alike) : DataTypeConversion  OutDataTypeStr=boolean
  Gain : Gain  Gain=1000
  Index Vector : MultiPortSwitch  DataPortOrder=Zero-based contiguous  Inputs=5  zeroidx=on
  MATLAB Function : MATLAB Function  TreatAsAtomicUnit=on
  MAV_FRAME_BODY_FRD : Constant  Value=8
  "MAV_FRAME_BODY_OFFSET_NED " : Constant  Value=9
  MAV_FRAME_LOCAL_NED : Constant
  "MAV_FRAME_LOCAL_NED " : Constant
  MAV_FRAME_LOCAL_OFFSET_NED : Constant  Value=7
  Mux : Mux  Inputs=2
  Mux1 : Mux
  Mux2 : Mux  Commented=on  Inputs=3
  Mux5 : Mux  Inputs=5
  Package Head : etargetslib/Byte Pack  Commented=on  datatypes={'uint32','int32'}  byteAlign=4
  TargetType : Constant  Commented=on  Value=3  OutDataTypeStr=Inherit: Inherit via back propagation
  len : Constant  Commented=on  Value=80  OutDataTypeStr=Inherit: Inherit via back propagation
  Out1 : Outport
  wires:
  Data Type Conversion7/1 -> MATLAB Function/5(Yaw)
  Data Type Conversion6/1 -> MATLAB Function/4(Force)
  vel/1 -> Mux5/2
  MAV_FRAME_BODY_FRD/1 -> Data Type Conversion11/1
  Data Type Conversion3/1 -> MATLAB Function/1(pos)
  Data Type Conversion5/1 -> MATLAB Function/3(Acc)
  Data Type Conversion4/1 -> MATLAB Function/2(vel)
  Data Type Conversion8/1 -> MATLAB Function/6(Yawrate)
  enAcc/1 -> Data Type Conversion5/1
  enYaw/1 -> Data Type Conversion7/1
  EnYawrate/1 -> Data Type Conversion8/1
  enForce/1 -> Data Type Conversion6/1
  "MAV_FRAME_LOCAL_NED "/1 -> Data Type Conversion9/1
  enPos/1 -> Data Type Conversion3/1
  Data Type Conversion9/1 -> Index Vector/2
  Data Type Conversion10/1 -> Index Vector/3
  Index Vector/1 -> Data Type Conversion/1  "coordinate_frame"
  Constant/1 -> Mux2/3  "uint8 (char) Payload[80:111]"
  Data Type Conversion18/1 -> Package Head/1
  Clock/1 -> Gain/1
  len/1 -> Data Type Conversion19/1
  Mux5/1 -> Mux/2
  MATLAB Function/1(y) -> Data Type Conversion1/1  "type_mask"
  Package Head/1 -> Mux2/1  "int (int32) TargetType & len"
  TargetType/1 -> Data Type Conversion18/1
  Gain/1 -> Mux1/1  "timestamp"
  Data Type Conversion19/1 -> Package Head/2
  pos/1 -> Mux5/1
  Byte Pack/1 -> Mux2/2  "uint8 (char) Payload[0:79]"
  Data Type Conversion13/1 -> Index Vector/6
  Data Type Conversion12/1 -> Index Vector/5
  acc/1 -> Mux5/3
  FrameIndex/1 -> Index Vector/1
  MAV_FRAME_LOCAL_NED/1 -> Data Type Conversion13/1
  MAV_FRAME_LOCAL_OFFSET_NED/1 -> Data Type Conversion10/1
  Data Type Conversion11/1 -> Index Vector/4
  "MAV_FRAME_BODY_OFFSET_NED "/1 -> Data Type Conversion12/1
  enVel/1 -> Data Type Conversion4/1
  yaw/1 -> Mux5/4
  yawrate/1 -> Mux5/5
  CopterID/1 -> Mux1/2
  Mux1/1 -> Mux/1
  Mux/1 -> Out1/1
  Data Type Conversion/1 -> Mux1/4
  Data Type Conversion1/1 -> Mux1/3

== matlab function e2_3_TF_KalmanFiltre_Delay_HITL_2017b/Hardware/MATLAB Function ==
function y = fcn(v,psi)

y = [v(1:2,1);-v(3);psi];

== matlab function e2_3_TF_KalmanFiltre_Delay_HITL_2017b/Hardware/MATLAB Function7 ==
function [x1,y1,h1,p1] = fcn(X,Y,H,Psi,t)

% position1=[u(1,1);u(3,1);0];
% position2=[u(2,1);u(4,1);0];
if t<5
    x1=0;
    y1=0;
    h1=-1;
    p1=0;
else
    x1=X;
    y1=Y;
    h1=-H;
    p1=Psi;
   
end

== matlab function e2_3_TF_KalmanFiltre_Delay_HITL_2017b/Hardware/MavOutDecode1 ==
function [Psi,localPos,localVel] = fcn(u)
localPos = [u(7:8);-u(9);u(6)];
localVel = u(10:12);
Psi=u(6);

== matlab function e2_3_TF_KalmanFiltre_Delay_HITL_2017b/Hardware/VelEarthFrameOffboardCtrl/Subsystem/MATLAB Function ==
function y = fcn(pos,vel,Acc,Force,Yaw,Yawrate)
y=uint32(0);
if ~pos
    y = bitor(y,uint32(7));
end

if~vel
    y = bitor(y,bitshift(uint32(7),3));
end

if ~Acc
    y = bitor(y,bitshift(uint32(7),6));
end

if Force
    y = bitor(y,bitshift(uint32(1),9));
end

if ~Yaw
    y = bitor(y,bitshift(uint32(1),10));
end

if ~Yawrate
    y = bitor(y,bitshift(uint32(1),11));
end

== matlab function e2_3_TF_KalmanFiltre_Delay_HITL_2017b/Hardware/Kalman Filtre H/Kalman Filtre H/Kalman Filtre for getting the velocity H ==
function [Covariance_matrice,X_Kalmanfiltred] = fcn(Mesurement_Velocity)

% Persistent process for saving the last state and initilizing the variable
persistent P0_static;
if isempty(P0_static)
    P0_static=[0.1,0 0;0,0.1,0;0 0 0.1]; % the initilized matrice of estimated error
end

persistent Xkf_static;
if isempty(Xkf_static)
    Xkf_static=[0;0;0]; % the initilized state from Kalman Estimaton
end

% Determine the constants

% Simple time
Ts =1/25;

% Process Noise
p_var =0.05; % sigma
Q = eye(3)*p_var^2; % the covariance matrice of process noise
W=Q*randn(3,1);  % process noise

% Mesurement Noise
m_var = 0.01; % sigma
R = [m_var^2 ];  % the covariance matrice of mesurement noise
V=R*randn; % mesurement noise

% Observation matrice
H=[1 0 0];

% The indentity matrice
I=eye(3); 

% State Transition Martrix
A=[1 Ts 0.5*(Ts^2);0 1 Ts;0 0 1];

% Steady-State equation

% persistent X_real_static;
% if isempty(X_real_static)
%     X_real_static=[0;0]; % the initilized state from Kalman Estimaton
% end
% X_real_forward=X_real_static;
% X_real=A*X_real_forward+W;
% Mesurement_Velocity=H*(X_real)+V;
% X_real_static=X_real;    

%   Kalman Update process
    X_pre=A*Xkf_static; % State estimation
    P_pre=A*P0_static*A'+Q; % Covariance matrice estimation

    Kg=P_pre*H'*inv(H*P_pre*H'+R); % Kalman Gain calculation

    X_Kalmanfiltred=X_pre+Kg*(Mesurement_Velocity-H*X_pre); % State estimation update
    Covariance_matrice=(I-Kg*H)*P_pre; % Covariance matrice estimation update

% update the value of the persistent variable for iterating the Kalman process
P0_static=Covariance_matrice;
Xkf_static=X_Kalmanfiltred;

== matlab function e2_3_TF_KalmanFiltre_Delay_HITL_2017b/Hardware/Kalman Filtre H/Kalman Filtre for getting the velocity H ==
function [Covariance_matrice,X_Kalmanfiltred] = fcn(Mesurement_Velocity) % Mesurement_State

% Persistent process for saving the last state and initilizing the variable
persistent P0_static;
if isempty(P0_static)
    P0_static=[[0.1,0 0;0,0.1,0;0 0 0.1] zeros(3) zeros(3) ;zeros(3) [0.1,0 0;0,0.1,0;0 0 0.1] zeros(3);zeros(3) zeros(3) [0.1,0 0;0,0.1,0;0 0 0.1]]; % the initilized matrice of estimated error
end

persistent Xkf_static;
if isempty(Xkf_static)
    Xkf_static=[0;0;0;0;0;0;0;0;0]; % the initilized state from Kalman Estimaton
end

% Determine the constants

% Simple time
Ts =1/25;

% Process Noise
p_var =0.1; % sigma
Q = eye(3)*p_var^2; % the covariance matrice of process noise
W=Q*randn(3,1);  % process noise
Q_delay=[Q zeros(3) zeros(3);zeros(3) Q zeros(3);zeros(3) zeros(3) Q];
% Mesurement Noise
m_var = 0.01; % sigma
R = [m_var^2 ];  % the covariance matrice of mesurement noise
V=R*randn; % mesurement noise
R_delay=R;
V_delay=R_delay*randn;
% Observation matrice
H=[1 0 0];
H_delay=[0 0 0 0 0 0 H];
% The indentity matrice
I=eye(3); 
I_delay=eye(9);

A=[1 Ts 0.5*(Ts^2);0 1 Ts;0 0 1];
A_delay=[A zeros(3) zeros(3);zeros(3) A zeros(3); zeros(3) zeros(3) A];
% Steady-State equation

% persistent X_real_static;
% if isempty(X_real_static)
%     X_real_static=[0;0]; % the initilized state from Kalman Estimaton
% end
% X_real_forward=X_real_static;
% X_real=A*X_real_forward+W;
% X_real_static=X_real;    
% Mesurement_Velocity=H_delay*(Mesurement_State)+V_delay;

%   Kalman Update process
    X_pre=A_delay*Xkf_static; % State estimation
    P_pre=A_delay*P0_static*A_delay'+Q_delay; % Covariance matrice estimation

    Kg=P_pre*H_delay'*inv(H_delay*P_pre*H_delay'+R_delay); % Kalman Gain calculation

    X_Kalmanfiltred=X_pre+Kg*(Mesurement_Velocity-H_delay*X_pre); % State estimation update
    Covariance_matrice=(I_delay-Kg*H_delay)*P_pre; % Covariance matrice estimation update

% update the value of the persistent variable for iterating the Kalman process
P0_static=Covariance_matrice;
Xkf_static=X_Kalmanfiltred;

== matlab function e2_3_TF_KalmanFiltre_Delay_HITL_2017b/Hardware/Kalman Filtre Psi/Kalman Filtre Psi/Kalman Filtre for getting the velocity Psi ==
function [Covariance_matrice,X_Kalmanfiltred] = fcn(Mesurement_Velocity)

% Persistent process for saving the last state and initilizing the variable
persistent P0_static;
if isempty(P0_static)
    P0_static=[0.1,0 0;0,0.1,0;0 0 0.1]; % the initilized matrice of estimated error
end

persistent Xkf_static;
if isempty(Xkf_static)
    Xkf_static=[0;0;0]; % the initilized state from Kalman Estimaton
end

% Determine the constants

% Simple time
Ts =1/25;

% Process Noise
p_var =0.01; % sigma
Q = eye(3)*p_var^2; % the covariance matrice of process noise
W=Q*randn(3,1);  % process noise

% Mesurement Noise
m_var = 0.05; % sigma
R = [m_var^2 ];  % the covariance matrice of mesurement noise
V=R*randn; % mesurement noise

% Observation matrice
H=[1 0 0];

% The indentity matrice
I=eye(3); 

% State Transition Martrix
A=[1 Ts 0.5*(Ts^2);0 1 Ts;0 0 1];


% Steady-State equation

% persistent X_real_static;
% if isempty(X_real_static)
%     X_real_static=[0;0]; % the initilized state from Kalman Estimaton
% end
% X_real_forward=X_real_static;
% X_real=A*X_real_forward+W;
% Mesurement_Velocity=H*(X_real)+V;
% X_real_static=X_real;    

%   Kalman Update process
    X_pre=A*Xkf_static; % State estimation
    P_pre=A*P0_static*A'+Q; % Covariance matrice estimation

    Kg=P_pre*H'*inv(H*P_pre*H'+R); % Kalman Gain calculation

    X_Kalmanfiltred=X_pre+Kg*(Mesurement_Velocity-H*X_pre); % State estimation update
    Covariance_matrice=(I-Kg*H)*P_pre; % Covariance matrice estimation update

% update the value of the persistent variable for iterating the Kalman process
P0_static=Covariance_matrice;
Xkf_static=X_Kalmanfiltred;

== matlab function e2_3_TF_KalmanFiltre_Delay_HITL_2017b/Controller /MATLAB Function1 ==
function [x,y] = fcn(eax,eay,psi)
g=9.8;

theta =eax/g;% vx
phi =eay/g;% vy
R=[cos(psi),-sin(psi);
    sin(psi),cos(psi)];
u=R^(-1)*[theta;phi];
x=u(1);
y=u(2);

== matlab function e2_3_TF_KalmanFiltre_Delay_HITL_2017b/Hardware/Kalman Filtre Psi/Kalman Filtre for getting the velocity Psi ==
function [Covariance_matrice,X_Kalmanfiltred] = fcn(Mesurement_Velocity) % Mesurement_State

% Persistent process for saving the last state and initilizing the variable
persistent P0_static;
if isempty(P0_static)
    P0_static=[[0.1,0 0;0,0.1,0;0 0 0.1] zeros(3) zeros(3) ;zeros(3) [0.1,0 0;0,0.1,0;0 0 0.1] zeros(3);zeros(3) zeros(3) [0.1,0 0;0,0.1,0;0 0 0.1]]; % the initilized matrice of estimated error
end

persistent Xkf_static;
if isempty(Xkf_static)
    Xkf_static=[0;0;0;0;0;0;0;0;0]; % the initilized state from Kalman Estimaton
end

% Determine the constants

% Simple time
Ts =1/25;

% Process Noise
p_var =0.05; % sigma
Q = eye(3)*p_var^2; % the covariance matrice of process noise
W=Q*randn(3,1);  % process noise
Q_delay=[Q zeros(3) zeros(3);zeros(3) Q zeros(3);zeros(3) zeros(3) Q];
% Mesurement Noise
m_var = 0.01; % sigma
R = [m_var^2 ];  % the covariance matrice of mesurement noise
V=R*randn; % mesurement noise
R_delay=R;
V_delay=R_delay*randn;
% Observation matrice
H=[1 0 0];
H_delay=[0 0 0 0 0 0 H];
% The indentity matrice
I=eye(3); 
I_delay=eye(9);

A=[1 Ts 0.5*(Ts^2);0 1 Ts;0 0 1];
A_delay=[A zeros(3) zeros(3);zeros(3) A zeros(3); zeros(3) zeros(3) A];
% Steady-State equation

% persistent X_real_static;
% if isempty(X_real_static)
%     X_real_static=[0;0]; % the initilized state from Kalman Estimaton
% end
% X_real_forward=X_real_static;
% X_real=A*X_real_forward+W;
% X_real_static=X_real;    
% Mesurement_Velocity=H_delay*(Mesurement_State)+V_delay;

%   Kalman Update process
    X_pre=A_delay*Xkf_static; % State estimation
    P_pre=A_delay*P0_static*A_delay'+Q_delay; % Covariance matrice estimation

    Kg=P_pre*H_delay'*inv(H_delay*P_pre*H_delay'+R_delay); % Kalman Gain calculation

    X_Kalmanfiltred=X_pre+Kg*(Mesurement_Velocity-H_delay*X_pre); % State estimation update
    Covariance_matrice=(I_delay-Kg*H_delay)*P_pre; % Covariance matrice estimation update

% update the value of the persistent variable for iterating the Kalman process
P0_static=Covariance_matrice;
Xkf_static=X_Kalmanfiltred;

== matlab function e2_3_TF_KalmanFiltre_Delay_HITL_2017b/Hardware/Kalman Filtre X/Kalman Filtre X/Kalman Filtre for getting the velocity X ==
function [Covariance_matrice,X_Kalmanfiltred] = fcn(Mesurement_Velocity)

% Persistent process for saving the last state and initilizing the variable
persistent P0_static;
if isempty(P0_static)
    P0_static=[0.1,0 0;0,0.1,0;0 0 0.1]; % the initilized matrice of estimated error
end

persistent Xkf_static;
if isempty(Xkf_static)
    Xkf_static=[0;0;0]; % the initilized state from Kalman Estimaton
end

% Determine the constants

% Simple time
Ts =1/25;

% Process Noise
p_var =0.05; % sigma
Q = eye(3)*p_var^2; % the covariance matrice of process noise
W=Q*randn(3,1);  % process noise

% Mesurement Noise
m_var = 0.01; % sigma
R = [m_var^2 ];  % the covariance matrice of mesurement noise
V=R*randn; % mesurement noise

% Observation matrice
H=[1 0 0];

% The indentity matrice
I=eye(3); 

% State Transition Martrix
A=[1 Ts 0.5*(Ts^2);0 1 Ts;0 0 1];

% Steady-State equation

% persistent X_real_static;
% if isempty(X_real_static)
%     X_real_static=[0;0]; % the initilized state from Kalman Estimaton
% end
% X_real_forward=X_real_static;
% X_real=A*X_real_forward+W;
% Mesurement_Velocity=H*(X_real)+V;
% X_real_static=X_real;    

%   Kalman Update process
    X_pre=A*Xkf_static; % State estimation
    P_pre=A*P0_static*A'+Q; % Covariance matrice estimation

    Kg=P_pre*H'*inv(H*P_pre*H'+R); % Kalman Gain calculation

    X_Kalmanfiltred=X_pre+Kg*(Mesurement_Velocity-H*X_pre); % State estimation update
    Covariance_matrice=(I-Kg*H)*P_pre; % Covariance matrice estimation update

% update the value of the persistent variable for iterating the Kalman process
P0_static=Covariance_matrice;
Xkf_static=X_Kalmanfiltred;
